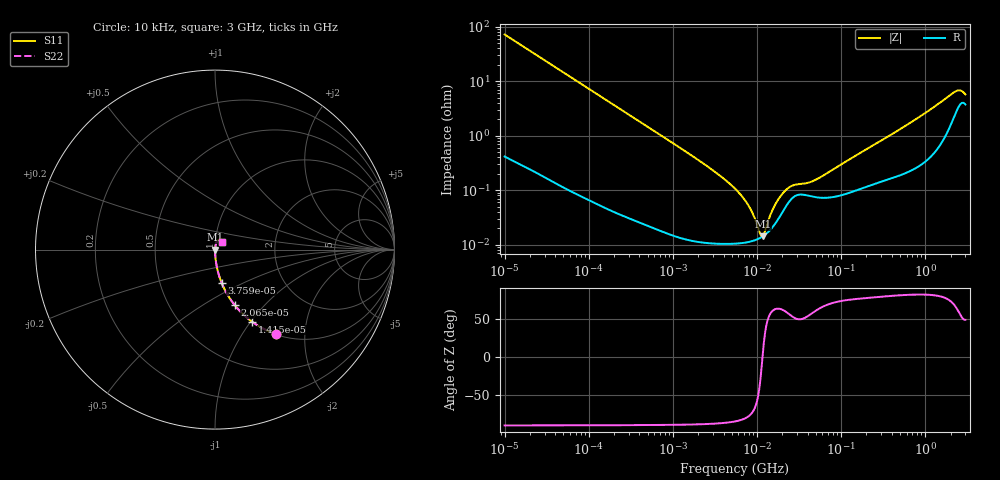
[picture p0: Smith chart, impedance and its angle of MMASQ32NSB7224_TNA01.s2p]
! MMASQ32NSB7224_TNA01  S-PARAMETER MODEL  ( Standard Model )
! Model Generated by TAIYO YUDEN Corporation (http://www.ty-top.com)
! Version 1.0
! TAIYO YUDEN Control No. 220601
! Copyright(c) 2013 TAIYO YUDEN CO.,LTD. All Rights Reserved.
! Product Description (link to TY-COMPAS)
! https://ds.yuden.co.jp/TYCOMPAS/or/detail?pn=MMASQ32NSB7224KTNA01&u=M
! Products Name : Multilayer Ceramic Capacitors
! Characteristics :
!  Capacitance : 0.22 [uF] , Rated Voltage : 250 [V] , TCC : X7R
!  Case Size : 3.2 x 2.5 / 0.126 x 0.098 [mm/inch] , Thickness : 1.9 / 0.075 [mm/inch]
!  (Conditions: Temperature = 25 [degC] , DC Bias Voltage = 0 [V])
! External Node Assignments :
!  1  o---| |---o  2
! GND o---------o GND
! Frequency Range : 10kHz  -  3GHz  [ 401 STEP ]
# MHZ S RI R 50
! Freq[MHz].  S11 Real  S11 Imag  S21 Real  S21 Imag  S12 Real  S12 Imag  S22 Real  S22 Imag
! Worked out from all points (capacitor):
!   401 points, 10 kHz to 3 GHz, reference 50 ohm
!   read as one part in series: C = 222 nF near 10.65 kHz
!   lowest |Z| = 14.1 mohm at 11.67 MHz (marker M1)
!   series resonance near 11.61 MHz, so ESL is about 850 pH
!   S11 on the Smith chart (normalised r, x): 10 kHz: 1.01, -1.43; 14.15 kHz: 1.01, -1.01; 20.65 kHz: 1.00, -0.70; 37.59 kHz: 1.00, -0.38; 3 GHz: 1.07, +0.09
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0.01  0.3401 -0.4709  0.6599 0.4709  0.6599 0.4709  0.3401 -0.4709
0.014146  0.2061 -0.4014  0.7939 0.4014  0.7939 0.4014  0.2061 -0.4014
0.020651  0.1096 -0.3091  0.8904 0.3091  0.8904 0.3091  0.1096 -0.3091
0.037592  0.0367 -0.1843  0.9633 0.1843  0.9633 0.1843  0.0367 -0.1843
0.082683  0.00832 -0.0866  0.9917 0.0866  0.9917 0.0866  0.00832 -0.0866
0.683653  0.000297 -0.0107  0.9997 0.0107  0.9997 0.0107  0.000297 -0.0107
2.737278  0.000112 -0.00255  0.9999 0.00255  0.9999 0.00255  0.000112 -0.00255
5.477226  0.000105 -0.00106  0.9999 0.00106  0.9999 0.00106  0.000105 -0.00106
7.996027  0.000112 -0.000497  0.9999 0.000497  0.9999 0.000497  0.000112 -0.000497
9.070798  0.000118 -0.000327  0.9999 0.000327  0.9999 0.000327  0.000118 -0.000327
10.95979  0.000133 -7.68e-05  0.9999 7.68e-05  0.9999 7.68e-05  0.000133 -7.68e-05
11.67315  0.000141 7.04e-06  0.9999 -7.04e-06  0.9999 -7.04e-06  0.000141 7.04e-06
12.43293  0.000151 9.18e-05  0.9998 -9.18e-05  0.9998 -9.18e-05  0.000151 9.18e-05
14.10408  0.00018 0.000265  0.9998 -0.000265  0.9998 -0.000265  0.00018 0.000265
15.99985  0.000228 0.000445  0.9998 -0.000445  0.9998 -0.000445  0.000228 0.000445
21.24962  0.000457 0.000832  0.9995 -0.000832  0.9995 -0.000832  0.000457 0.000832
26.49725  0.000722 0.000975  0.9993 -0.000975  0.9993 -0.000975  0.000722 0.000975
45.28751  0.000762 0.00123  0.9992 -0.00123  0.9992 -0.00123  0.000762 0.00123
374.4521  0.00169 0.00979  0.9983 -0.00979  0.9983 -0.00979  0.00169 0.00979
2188.735  0.0242 0.0557  0.9758 -0.0557  0.9758 -0.0557  0.0242 0.0557
2562.461  0.0379 0.0533  0.9621 -0.0533  0.9621 -0.0533  0.0379 0.0533
3000  0.0375 0.0403  0.9625 -0.0403  0.9625 -0.0403  0.0375 0.0403
